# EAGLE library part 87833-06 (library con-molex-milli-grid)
HEADER
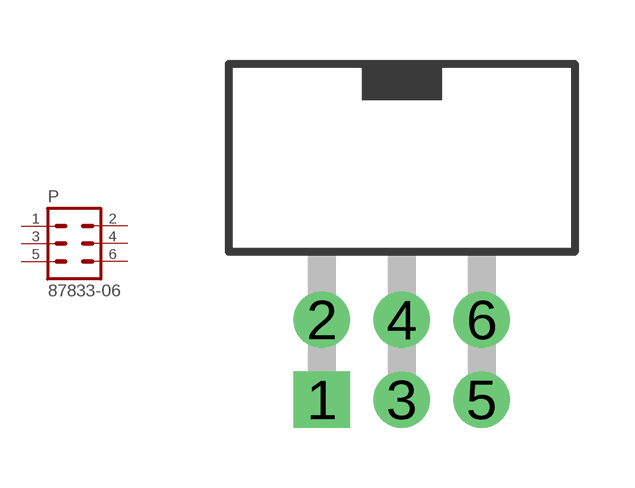
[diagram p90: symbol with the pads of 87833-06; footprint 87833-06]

Designator prefix P

## 87833-06  [87833-06]
1  1  pas
2  2  pas
3  3  pas
4  4  pas
5  5  pas
6  6  pas

## Footprint 87833-06 (pad centres in mm)
HEADER Dual Row, Shrouded, Right Angle
drill 0.914 square: 1 -2,-1
drill 0.914: 2 -2,1; 3 0,-1; 4 0,1; 5 2,-1; 6 2,1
